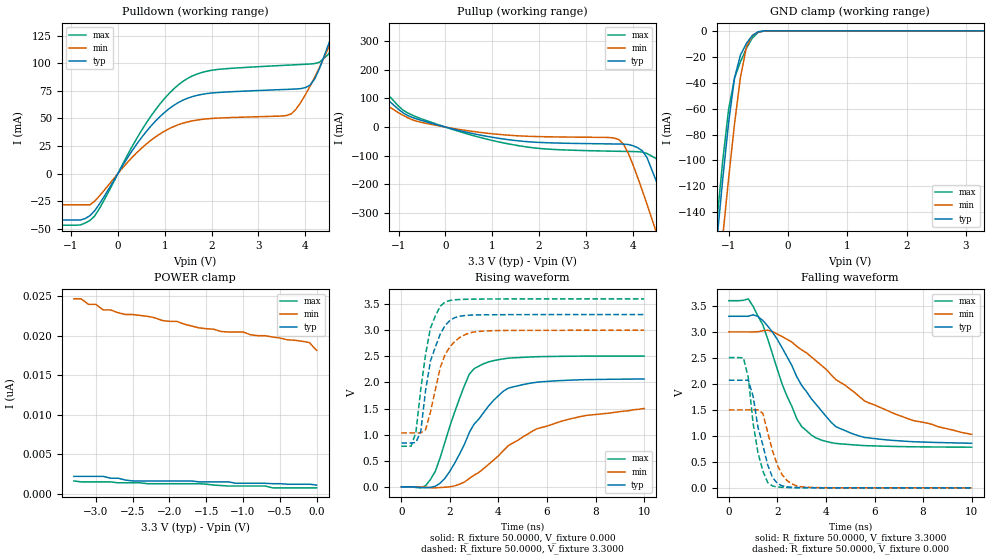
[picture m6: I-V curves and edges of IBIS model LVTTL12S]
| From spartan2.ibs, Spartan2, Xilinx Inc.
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|   Model LVTTL12S
[Model]   LVTTL12S
Model_type   I/O
Polarity   Non-Inverting
Enable   Active-Low
Vinl =   0.800V
Vinh =   2.000V
Vmeas =   1.4000V
Cref =  35.0000pF
Rref =   1.0000M
Vref =  0.000V
C_comp   6.5000pF   5.0000pF   8.0000pF
[Temperature Range]   27.0000   100.0000   0.000
[Voltage Range]   3.3000V   3.0000V   3.6000V
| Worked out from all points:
|   slope of the pulldown table from 0 to 0.495 V, typ, clamps not added: 15.4 ohm
|   slope of the pullup table from 0 to 0.495 V, typ, clamps not added: 25.2 ohm
|   GND clamp passes 1 mA (typ) near -0.51 V on its own axis
|   rising waveform, R_fixture 50.0000, V_fixture 0.000: 20-80 % time 1.65ns typ, 2.99ns min, 1.11ns max; typ from 0 V to 2.06 V
|   rising waveform, R_fixture 50.0000, V_fixture 3.3000: 20-80 % time 638ps typ, 706ps min, 524ps max; typ from 0.84 V to 3.3 V
|   falling waveform, R_fixture 50.0000, V_fixture 3.3000: 20-80 % time 2.01ns typ, 3.68ns min, 1.31ns max; typ from 3.3 V to 0.859 V
|   falling waveform, R_fixture 50.0000, V_fixture 0.000: 20-80 % time 589ps typ, 618ps min, 473ps max; typ from 2.07 V to 0 V
[Pulldown]
| voltage   I(typ)   I(min)   I(max)
-3.3V     -42.12mA   -28.36mA   -46.83mA
-600mV    -38.25mA   -28.36mA   -42.6mA
-400mV    -27.87mA   -20.58mA   -32.11mA
700mV     42.79mA    29.97mA    51.76mA
1.2V      61.98mA    42.74mA    77.02mA
1.6V      69.81mA    47.81mA    88.61mA
3.7V      76.41mA    54.11mA    98.37mA
4.1V      80.11mA    79.08mA    99.25mA
4.3V      94.94mA    96.03mA    100.8mA
4.5V      117.6mA    114.4mA    108.3mA
4.7V      142.5mA    133.7mA    132.4mA
6.6V      399mA      330.4mA    441.4mA
[Pullup]
| voltage   I(typ)   I(min)   I(max)
-3.3V     401.3mA    308.2mA    484mA
-2.9V     344.8mA    263.9mA    415.5mA
-2.5V     286.5mA    217.5mA    345.7mA
-700mV    33.24mA    24.98mA    41.08mA
1.5V      -47.01mA   -30.01mA   -63.27mA
3.7V      -59.11mA   -43.53mA   -84.54mA
3.9V      -60.79mA   -90.24mA   -85.1mA
4.2V      -82.34mA   -220.4mA   -87.26mA
4.5V      -188.3mA   -366.3mA   -110.2mA
4.9V      -390.3mA   -567.2mA   -235.3mA
5.1V      -496mA     -668.9mA   -335.5mA
6.6V      -1.307A    -1.44A     -1.153A
[GND_clamp]
| voltage   I(typ)   I(min)   I(max)
-3.3V     -1.286A    -1.273A    -1.289A
-1.2V     -163.3mA   -206.7mA   -148.3mA
-1.1V     -115.2mA   -159.6mA   -101mA
-1V       -71.04mA   -114.2mA   -60.78mA
-900mV    -36.42mA   -71.86mA   -36.53mA
-800mV    -18.72mA   -35.86mA   -23.84mA
-700mV    -9.715mA   -12.62mA   -13.63mA
-600mV    -3.608mA   -3.649mA   -5.602mA
-500mV    -692.7uA   -854.2uA   -1.156mA
-400mV    -68.48uA   -138.7uA   -98.54uA
-300mV    -4.365uA   -16.73uA   -4.627uA
3.3V      1.048nA    19.44nA    40.34nA
[POWER_clamp]
| voltage   I(typ)   I(min)   I(max)
-3.3V     2.212nA    24.68nA    1.63nA
-3.2V     2.212nA    24.68nA    1.513nA
-3.1V     2.212nA    23.98nA    1.513nA
-3V       2.212nA    23.98nA    1.513nA
-2.9V     2.212nA    23.28nA    1.513nA
-2.6V     1.746nA    22.7nA     1.397nA
-1.9V     1.63nA     21.83nA    1.281nA
-1.3V     1.513nA    20.55nA    1.048nA
-1V       1.339nA    20.49nA    989.5pA
-900mV    1.339nA    20.14nA    989.5pA
-100mV    1.222nA    19.15nA    756.7pA
0V        1.106nA    18.16nA    756.7pA
[Ramp]
| variable   typ   min   max
dV/dt_r   1.2390/1.6423n   0.8730/2.7720n   1.5030/1.0990n
dV/dt_f   1.4647/2.0141n   1.1166/3.2951n   1.6905/1.3442n
R_load = 50.0000
[Rising Waveform]
R_fixture = 50.0000
V_fixture = 0.000
| time   V(typ)   V(min)   V(max)
0s        0V         0V         0V
800ps     -11.64mV   901.8uV    -16.88mV
1.2ns     -7.903mV   -14.23mV   141.6mV
2ns       301.5mV    2.076mV    1.165V
2.6ns     817mV      94.13mV    1.94V
3ns       1.205V     226.1mV    2.264V
4ns       1.747V     595.7mV    2.434V
4.6ns     1.914V     842.5mV    2.47V
6.8ns     2.041V     1.284V     2.501V
10ns      2.065V     1.502V     2.505V
[Rising Waveform]
R_fixture = 50.0000
V_fixture = 3.3000
V_fixture_min = 3.0000
V_fixture_max = 3.6000
| time   V(typ)   V(min)   V(max)
0s        840.3mV    1.034V     778.4mV
400ps     840.8mV    1.034V     779.6mV
600ps     850.7mV    1.034V     1.043V
800ps     1.063V     1.034V     1.867V
1ns       1.853V     1.094V     2.54V
1.2ns     2.411V     1.435V     3.043V
1.6ns     2.922V     2.281V     3.457V
1.8ns     3.087V     2.53V      3.538V
3ns       3.291V     2.966V     3.594V
10ns      3.299V     2.999V     3.599V
[Falling Waveform]
R_fixture = 50.0000
V_fixture = 3.3000
V_fixture_min = 3.0000
V_fixture_max = 3.6000
| time   V(typ)   V(min)   V(max)
0s        3.3V       3V         3.6V
800ps     3.301V     3V         3.635V
1ns       3.329V     2.999V     3.491V
1.4ns     3.219V     3.022V     3.136V
1.8ns     2.993V     3.006V     2.571V
2.8ns     2.135V     2.722V     1.327V
3.6ns     1.603V     2.441V     958.1mV
4.4ns     1.18V      2.084V     854.7mV
5.6ns     969.4mV    1.669V     812.4mV
10ns      858.8mV    1.029V     782.5mV
[Falling Waveform]
R_fixture = 50.0000
V_fixture = 0.000
| time   V(typ)   V(min)   V(max)
0s        2.07V      1.5V       2.506V
600ps     2.07V      1.5V       2.501V
800ps     2.072V     1.5V       2.126V
1ns       1.762V     1.5V       1.24V
1.2ns     1.164V     1.501V     675.7mV
1.4ns     824.4mV    1.431V     329.3mV
1.8ns     198.6mV    710.9mV    36.27mV
2.2ns     37.73mV    249.9mV    9.903mV
2.8ns     6.475mV    36.61mV    3.539mV
10ns      341.4uV    468.3uV    303.9uV
